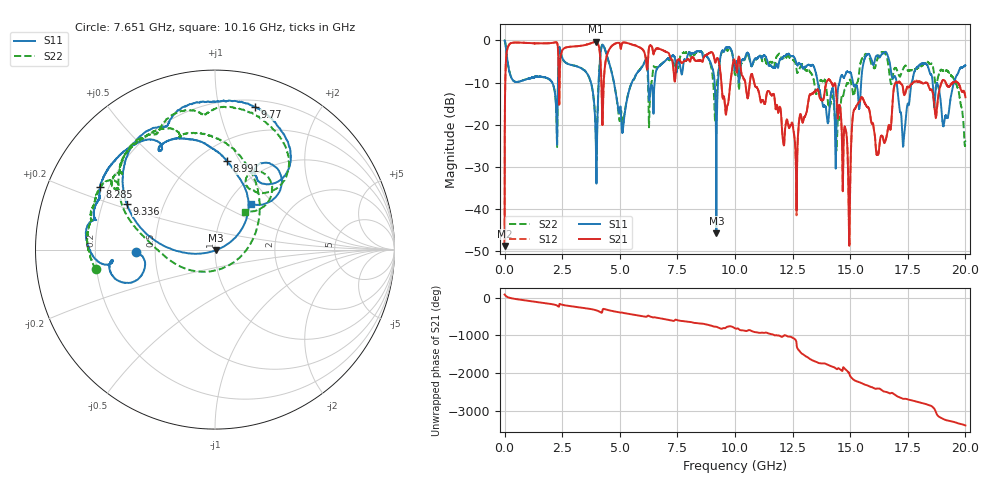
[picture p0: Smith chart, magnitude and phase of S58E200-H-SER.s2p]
!{S58E200}
!Johanson Technology Inc.
!www.johansontechnology.com
!Test Board Conditions:
!Substrate Type  RO4350B
!Substrate Thickness  60 mil
!Substrate Dk  3.66
!TL Type: GCPW
!TL Trace Width  115 mil
!TL Gap  52 mil
!Electrode orientation  Horizontal
!DUT TOPOLOGY	SERIES
!Mounting Pad LxW  55x428 mil
! Created Wed Apr 14 11:26:49 2021
# mhz S ma R 50
! 2 Port Network Data from SP1.SP block
! freq  magS11  angS11  magS21  angS21  magS12  angS12  magS22  angS22
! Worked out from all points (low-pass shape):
!   20001 points, 300 kHz to 20 GHz, reference 50 ohm
!   highest |S21| = -0.32 dB at 3.963 GHz (marker M1); lowest = -48.8 dB at 300 kHz (marker M2)
!   |S21| within 3 dB of the highest: 80.42 MHz to 2.327 GHz (2.246 GHz wide, 187 % of centre); 2.448 GHz to 4.141 GHz (1.694 GHz wide, 51.4 % of centre)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
!   lowest |S11| = -45.8 dB at 9.189 GHz (marker M3), VSWR 1.01, Z = 50.4 - j0.36 ohm
!   |S11| at or under -10 dB: 4.748 GHz to 5.523 GHz (775.4 MHz wide, 15.1 % of centre); 13.59 GHz to 14.54 GHz (943.7 MHz wide, 6.71 % of centre); 18.58 GHz to 19.5 GHz (918.8 MHz wide, 4.83 % of centre)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
!   |S22| runs from -28.5 to 0.0 dB; largest |S21 - S12| = 0.0094
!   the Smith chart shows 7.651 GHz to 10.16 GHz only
!   S11 on the Smith chart (normalised r, x): 7.651 GHz: 0.39, -0.01; 8.285 GHz: 0.17, +0.25; 8.991 GHz: 0.67, +0.89; 9.336 GHz: 0.30, +0.22; 9.77 GHz: 0.26, +1.29; 10.16 GHz: 1.28, +0.72
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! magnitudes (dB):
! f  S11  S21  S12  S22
! 300 kHz  0.0  -48.8  -48.9  0.0
! 208.3 MHz  -7.4  -0.9  -0.9  -7.4
! 3.334 GHz  -6.6  -1.2  -1.2  -6.6
! 3.963 GHz  -25.1  -0.3  -0.3  -24.1
! 4.262 GHz  -1.0  -17.2  -17.2  -1.0
! 5.137 GHz  -21.1  -0.5  -0.5  -19.3
! 6.667 GHz  -6.4  -1.9  -1.9  -6.2
! 7.651 GHz  -7.2  -5.2  -5.2  -3.4
! 8.285 GHz  -2.8  -4.8  -4.8  -3.0
! 8.991 GHz  -6.0  -2.8  -2.8  -7.0
! 9.189 GHz  -45.8  -4.6  -4.6  -12.2
! 9.336 GHz  -5.1  -6.2  -6.2  -4.8
! 9.77 GHz  -1.7  -11.6  -11.6  -2.0
! 10 GHz  -6.9  -5.1  -5.1  -8.1
! 10.16 GHz  -9.8  -3.8  -3.8  -11.4
! 12.64 GHz  -5.1  -30.1  -30.1  -5.9
! 13.33 GHz  -5.8  -12.7  -12.6  -8.0
! 14.95 GHz  -7.5  -47.2  -46.2  -9.7
! 15.43 GHz  -14.4  -14.3  -14.3  -5.7
! 16.67 GHz  -4.3  -20.3  -20.1  -6.3
! 17.32 GHz  -23.9  -12.5  -12.4  -6.5
! 20 GHz  -5.9  -13.5  -13.3  -23.9
